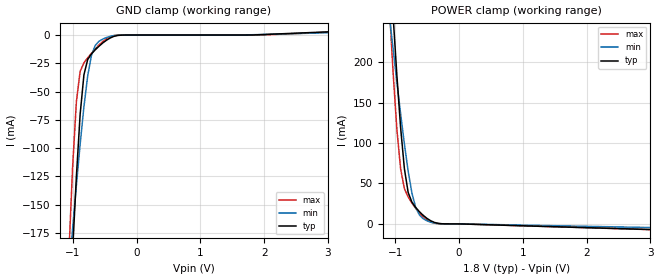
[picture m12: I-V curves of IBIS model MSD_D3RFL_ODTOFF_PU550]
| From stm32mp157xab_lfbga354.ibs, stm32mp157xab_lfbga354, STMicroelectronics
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[Model] MSD_D3RFL_ODTOFF_PU550
Model_type   Input
C_comp 2.381pF   2.320pF   2.527pF
Vinh = 1.440V
Vinl = 360.000mV
[Temperature Range]   25.000   125.000   -40.000
[Voltage Range]   1.800V   1.650V   1.950V
[GND Clamp Reference]   0.00V   0.00V   0.00V
[POWER Clamp Reference]   1.800V   1.650V   1.950V
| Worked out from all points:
|   GND clamp passes 1 mA (typ) near -0.34 V on its own axis
|   POWER clamp passes 1 mA (typ) near -0.35 V on its own axis
[GND Clamp]
-1.773V   -1.216A    -713mA     -1.315A
-1.064V   -264.3mA   -211.2mA   -194.3mA
-1.005V   -191.7mA   -171.5mA   -117.3mA
-945.5mV  -125.1mA   -133.1mA   -59.1mA
-886.4mV  -70.08mA   -96.59mA   -32.01mA
-827.3mV  -35.23mA   -63.55mA   -24.64mA
-768.2mV  -21.73mA   -36.24mA   -20.21mA
-709.1mV  -16.67mA   -17.95mA   -16.15mA
-650mV    -13.09mA   -9.203mA   -12.34mA
-531.8mV  -7.03mA    -3.571mA   -5.757mA
-236.4mV  -77.02uA   -35.01uA   -8.019uA
3.545V    4.093mA    2.883mA    3.802mA
[Power Clamp]
-1.745V   1.222A     726.4mA    1.305A
-1.095V   334.1mA    257.5mA    268.6mA
-1.036V   257.3mA    216.3mA    187mA
-977.3mV  184.1mA    175.7mA    117.2mA
-918.2mV  119mA      136.3mA    68.02mA
-859.1mV  68.3mA     98.87mA    43.69mA
-800mV    38.82mA    65.22mA    33.27mA
-740.9mV  26.87mA    38.1mA     25.75mA
-681.8mV  20.3mA     20.25mA    19.19mA
-563.6mV  10.53mA    6.418mA    8.675mA
-268.2mV  165.1uA    101.6uA    32.81uA
3.573V    -8.289mA   -5.357mA   -8.46mA
